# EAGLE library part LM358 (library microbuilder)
LM358 Dual Operational Amplifier Digikey: LM358AMXFSCT-ND
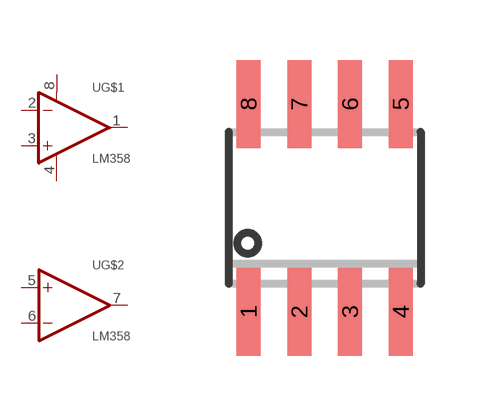
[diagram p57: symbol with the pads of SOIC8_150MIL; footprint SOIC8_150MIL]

Designator prefix U; gates G$1=OPAMP+- G$2=OPAMP

## LM358  [SOIC8_150MIL]
1  G$1:OUT  out
2  G$1:-IN  in
3  G$1:+IN  in
4  G$1:V-  pwr
5  G$2:+IN  in
6  G$2:-IN  in
7  G$2:OUT  out
8  G$1:V+  pwr

## Footprint SOIC8_150MIL (pad centres in mm)
Small Outline IC - 150mil Wide
smd 0.6 x 2.2: 1 -1.905,-2.6; 2 -0.635,-2.6; 3 0.635,-2.6; 4 1.905,-2.6; 5 1.905,2.6; 6 0.635,2.6; 7 -0.635,2.6; 8 -1.905,2.6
